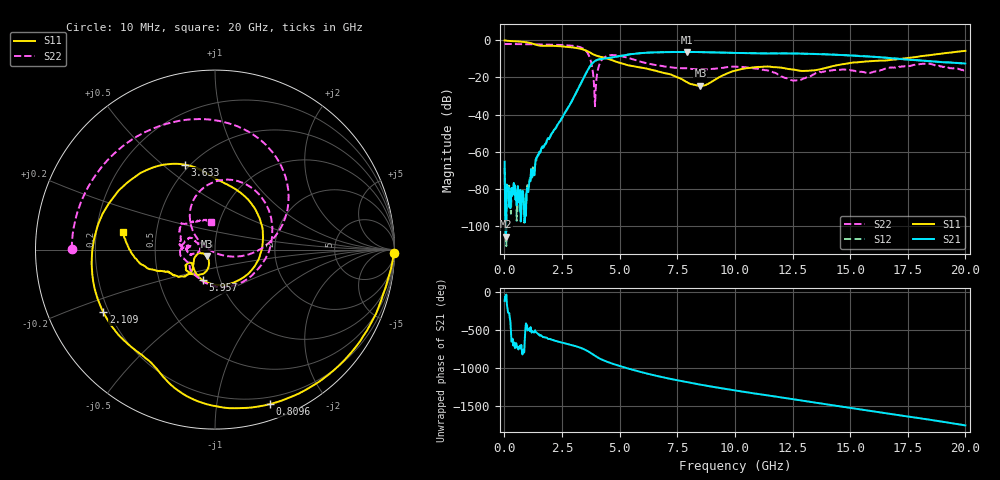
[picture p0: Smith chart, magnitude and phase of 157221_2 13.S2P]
!  2-Port S-parameters saved by WinCal
! VAR MeasName=S-Parameters (CALIBRATED_DATA) read from VNA (N5242A)
! VAR MeasDate=2015-5-26 16:48:00
! VAR NAME=157221_2 13
! VAR FILENAME=157221_2 13.S2P
! VAR DATE=2015-5-26 16:48:00
! VAR PHYS_PORTS=1,2
# Hz S DB R 50
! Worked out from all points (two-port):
!   801 points, 10 MHz to 20 GHz, reference 50 ohm
!   highest |S21| = -6.20 dB at 7.906 GHz (marker M1); lowest = -105.9 dB at 59.98 MHz (marker M2)
!   |S21| within 3 dB of the highest: 4.672 GHz to 16.45 GHz (11.78 GHz wide, 112 % of centre)
!   lowest |S11| = -24.5 dB at 8.506 GHz (marker M3), VSWR 1.13, Z = 45.4 - j3.42 ohm
!   |S11| at or under -10 dB: 4.512 GHz to 17.17 GHz (12.66 GHz wide, 117 % of centre)
!   |S22| runs from -35.5 to -2.0 dB; largest |S21 - S12| = 0.01
!   S11 on the Smith chart (normalised r, x): 10 MHz: open; 809.6 MHz: 0.14, -1.41; 2.109 GHz: 0.18, -0.25; 3.633 GHz: 0.47, +0.60; 5.957 GHz: 0.83, -0.29; 20 GHz: 0.32, +0.09
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1e7  -0.04 -1.1  -65.38 -115.6  -68.66 150.9  -1.96 179.8
5.9975e7  -0.12 -6.3  -105.88 -75.9  -95.32 -163.3  -1.96 178.5
1.349375e8  -0.24 -12.9  -80.20 139.8  -81.79 132.0  -1.96 176.6
8.096e8  -0.78 -70.4  -81.24 -40.6  -84.79 -23.5  -2.02 160.4
2.10895e9  -2.93 -150.8  -49.51 87.4  -49.38 87.2  -2.32 124.5
3.358325e9  -4.68 130.4  -22.29 -21.7  -22.27 -22.1  -4.00 59.6
3.633188e9  -6.00 109.4  -15.65 -62.3  -15.65 -62.7  -7.29 24.7
3.933038e9  -7.94 90.6  -11.07 -121.3  -11.09 -121.5  -35.47 -135.0
4.157925e9  -8.81 76.2  -10.10 -160.9  -10.11 -161.0  -11.91 123.3
4.432788e9  -9.71 52.1  -9.66 162.6  -9.65 162.5  -8.51 91.4
5.2074e9  -12.83 -37.0  -7.98 85.3  -7.96 85.0  -8.86 30.5
5.957025e9  -14.73 -111.9  -6.82 21.7  -6.82 21.4  -11.68 -26.1
6.681662e9  -16.80 -146.1  -6.36 -31.6  -6.36 -31.8  -13.45 -80.9
7.90605e9  -22.41 -164.4  -6.20 -108.3  -6.21 -108.6  -15.05 -141.2
8.50575e9  -24.47 -141.2  -6.30 -142.5  -6.30 -142.7  -15.62 -150.6
1.0005e10  -16.29 -116.9  -6.75 141.3  -6.74 140.9  -14.19 -173.8
1.152924e10  -14.15 -146.0  -7.03 70.7  -7.02 70.2  -16.63 153.7
1.335332e10  -16.22 -143.2  -7.31 -13.8  -7.27 -14.1  -18.75 -169.0
1.492754e10  -12.36 -141.9  -8.10 -86.6  -8.04 -86.7  -15.97 172.8
1.667666e10  -10.67 -155.3  -9.48 -166.9  -9.49 -167.2  -14.72 178.5
1.837581e10  -8.07 -165.4  -11.17 117.5  -11.09 116.2  -12.45 142.4
2e10  -5.65 168.9  -12.47 38.4  -12.52 36.7  -16.21 97.5
